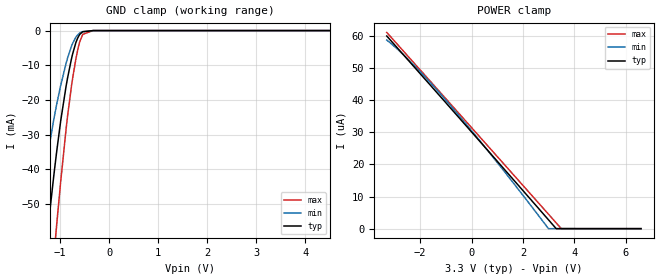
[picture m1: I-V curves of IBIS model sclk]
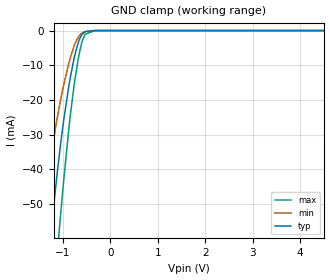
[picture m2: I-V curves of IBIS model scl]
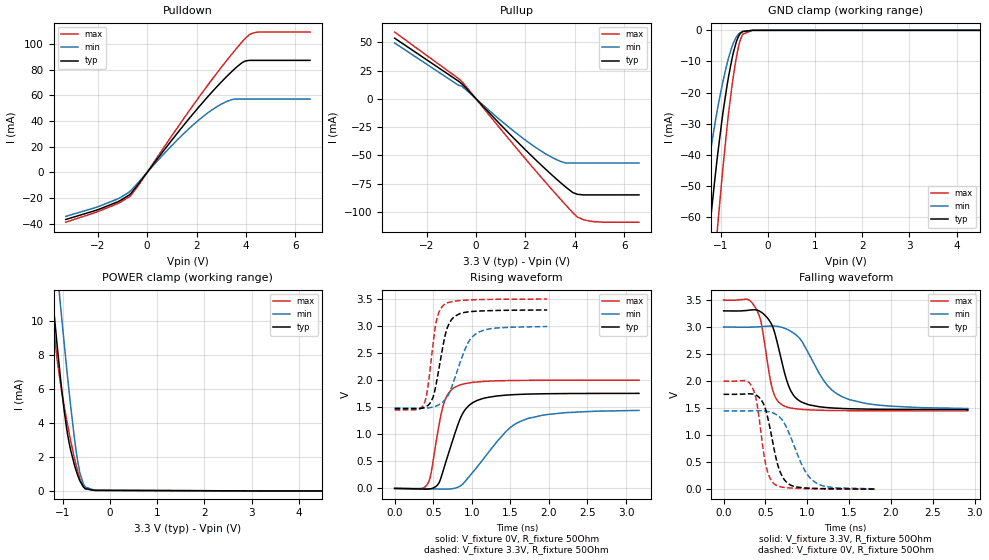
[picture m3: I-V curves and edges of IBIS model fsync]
|Texas Instruments Incorporated
|50-W, 2-MHz Digital Input 4-Channel Automotive Class-D Audio Amplifier
|With Load Dump Protection and I2C Diagnostics
|Marketing part#   Digital Voltage Range   Package-type   #pins
|TAS6424-Q1   3V - 26.4V   HSSOP   56
[IBIS Ver]   4.1
[File name]   tas6424_q1.ibs
[File Rev]   1.0
[Date]   9/17/2016
[Source]
| Texas Instruments Incorporated.
| Analog-eLab Design Center, HPA
| 12500 TI Blvd
| Dallas, TX -75243
[Notes]   Revision History:
| Rev 1.0: 9/17/2016
| - Initial version of the model
| - Model generated from simulations in SPECTRE
| - Model matched to SPICE simulation
| - C_comp although listed in numerical order of value are
|   obtained from varying PVT conditions. For PVT conditions for
|   each specific value refer the buffer description under
|   respective [Model]. IBIS model user is responsible for using
|   appropriate C_comp to simulate for Signal Integrity.
[Disclaimer]
| This model is designed as an aid for customers of Texas Instruments.
| TI and its licensors and suppliers make no warranties, either expressed
| or implied, with respect to this  model, including the warranties of
| merchantability or fitness for a particular purpose. The model is
| provided solely on an "as is" basis. The entire risk as to its quality
| and performance is with the customer.
[Copyright]
(C) Copyright 2016 Texas Instruments Incorporated.All rights reserved.
|   TAS6424_Q1DKQ
[Component]   TAS6424_Q1DKQ
[Manufacturer]   TI
[Package]   |56 DKQ - HSSOP Package
|   typ   min   max
R_pkg   0.2   0.16   0.24
L_pkg   1.5nH   1.2nH   1.8nH
C_pkg   0.4pF   0.32pF   0.48pF
[Pin]  signal_name   model_name   R_pin   L_pin   C_pin
1   GND   gnd   NA   NA   NA
2   PVDD   power   NA   NA   NA
3   VBAT   power   NA   NA   NA
4   AREF   power   NA   NA   NA
5   VREG   power   NA   NA   NA
6   VCOM   power   NA   NA   NA
7   AVSS   power   NA   NA   NA
8   AVDD   power   NA   NA   NA
9   GVDD   power   NA   NA   NA
10   GVDD   power   NA   NA   NA
11   GND   gnd   NA   NA   NA
12   MCLK   sclk   NA   NA   NA
13   SCLK   sclk   NA   NA   NA
14   FSYNC   fsync   NA   NA   NA
15   SDIN1   sclk   NA   NA   NA
16   SDIN2   sclk   NA   NA   NA
17   GND   gnd   NA   NA   NA
18   GND   gnd   NA   NA   NA
19   VDD   power   NA   NA   NA
20   SCL   scl   NA   NA   NA
21   SDA   sda   NA   NA   NA
22   I2C_ADDR0   fsync   NA   NA   NA
23   I2C_ADDR1   fsync   NA   NA   NA
24   _STANDBY   nc   NA   NA   NA
25   _MUTE   nc   NA   NA   NA
26   _FAULT   nc   NA   NA   NA
27   _WARN   nc   NA   NA   NA
28   GND   nc   NA   NA   NA
29   PVDD   power   NA   NA   NA
30   PVDD   power   NA   NA   NA
31   BST_1M   power   NA   NA   NA
32   OUT_1M   nc   NA   NA   NA
33   GND   gnd   NA   NA   NA
34   OUT_1P   nc   NA   NA   NA
35   BST_1P   power   NA   NA   NA
36   GND   gnd   NA   NA   NA
37   BST_2M   power   NA   NA   NA
38   OUT_2M   nc   NA   NA   NA
39   GND   gnd   NA   NA   NA
40   OUT_2P   nc   NA   NA   NA
41   BST_2P   power   NA   NA   NA
42   PVDD   power   NA   NA   NA
43   PVDD   power   NA   NA   NA
44   BST_3M   power   NA   NA   NA
45   OUT_3M   nc   NA   NA   NA
46   GND   gnd   NA   NA   NA
47   OUT_3P   nc   NA   NA   NA
48   BST_3P   power   NA   NA   NA
49   GND   gnd   NA   NA   NA
50   BST_4M   power   NA   NA   NA
51   OUT_4M   nc   NA   NA   NA
52   GND   gnd   NA   NA   NA
53   OUT_4P   nc   NA   NA   NA
54   BST_4P   power   NA   NA   NA
55   PVDD   power   NA   NA   NA
56   PVDD   power   NA   NA   NA
57   ThermalPad   gnd   NA   NA   NA
| Models and submodels in the file (4): sclk (Input), scl (Input), fsync (I/O), sda (I/O_open_drain)
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|   sclk Model
[Model]   sclk
Model_type   Input
Vinl = 0.99
Vinh = 2.31
|   typ   min   max
|   (nom PVT)   (fast PVT)   (slow PVT)
C_comp   6.288e-13   4.758e-13   7.537e-13
| Where nom  PVT is Nominal Process, 3.3V, 27C
|   Fast PVT is Strong Process,  3.5V, -40C
|   Slow PVT is Weak Process,   3V, 150C
[Model spec]
|subparameter
Vinl   0.99   0.90   1.05
Vinh   2.31   2.10   2.45
[Voltage Range]   3.3   3   3.5
|Junction Temperature
[Temperature Range]   27   150   -40
[Power Clamp Reference]   3.3   3   3.5
[GND Clamp Reference]   0   0   0
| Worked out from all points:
|   GND clamp passes 1 mA (typ) near -0.59 V on its own axis
[GND Clamp]
|   Voltage   I(typ)   I(min)   I(max)
-3.3V     -394.6mA   -304mA     -465.7mA
-1.544V   -99.89mA   -64.75mA   -138.1mA
-1.449V   -85.57mA   -54.72mA   -120.8mA
-1.287V   -62.45mA   -39.03mA   -92.13mA
-1.238V   -55.77mA   -34.62mA   -83.61mA
-1.105V   -39.1mA    -23.91mA   -61.71mA
-1.067V   -34.61mA   -21.1mA    -55.6mA
-877.8mV  -16.02mA   -9.455mA   -28.4mA
-769.5mV  -8.244mA   -4.559mA   -16.14mA
-642mV    -2.163mA   -1.241mA   -5.637mA
-538.5mV  -332.8uA   -295.2uA   -1.103mA
6.6V      0A         0A         0A
[POWER Clamp]
|   Voltage   I(typ)   I(min)   I(max)
-3.3V     59.92uA    58.65uA    61.04uA
-2.808V   55.49uA    55.28uA    56.63uA
-2.225V   50.24uA    50.72uA    51.41uA
-1.455V   43.28uA    44.1uA     44.5uA
-801mV    37.36uA    38.12uA    38.63uA
1.005V    20.95uA    20.55uA    22.41uA
2.997V    2.746uA    0A         4.496uA
3.297V    0A         0A         1.799uA
3.495V    0A         0A         17.75nA
6.6V      0A         0A         0A
|   scl Model
[Model]   scl
Model_type   Input
Vinl = 0.99
Vinh = 2.31
|   typ   min   max
|   (nom PVT)   (fast PVT)   (slow PVT)
C_comp   6.288e-13   4.758e-13   7.537e-13
| Where nom  PVT is Nominal Process, 3.3V, 27C
|   Fast PVT is Strong Process,  3.5V, -40C
|   Slow PVT is Weak Process,   3V, 150C
[Model spec]
|subparameter
Vinl   0.99   0.90   1.05
Vinh   2.31   2.10   2.45
[Voltage Range]   3.3   3   3.5
|Junction Temperature
[Temperature Range]   27   150   -40
[Power Clamp Reference]   3.3   3   3.5
[GND Clamp Reference]   0   0   0
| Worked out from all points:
|   GND clamp passes 1 mA (typ) near -0.59 V on its own axis
[GND Clamp]
|   Voltage   I(typ)   I(min)   I(max)
-3.3V     -394.6mA   -304mA     -465.7mA
-1.544V   -99.89mA   -64.75mA   -138.1mA
-1.449V   -85.57mA   -54.72mA   -120.8mA
-1.287V   -62.45mA   -39.03mA   -92.13mA
-1.238V   -55.77mA   -34.62mA   -83.61mA
-1.105V   -39.09mA   -23.91mA   -61.71mA
-1.067V   -34.61mA   -21.1mA    -55.6mA
-877.8mV  -16.02mA   -9.452mA   -28.4mA
-769.5mV  -8.242mA   -4.556mA   -16.14mA
-642mV    -2.16mA    -1.238mA   -5.635mA
-538.5mV  -329.1uA   -291.4uA   -1.101mA
6.6V      0A         0A         0A
[POWER Clamp]
|   Voltage   I(typ)   I(min)   I(max)
-3.3V     0A         0A         0A
0V        0A         0A         0A
6.6V      0A         0A         0A
|   fsync Model
[Model]   fsync
Model_type   I/O
Polarity   Non-Inverting
Enable   Active-High
Vinl = 0.99
Vinh = 2.31
Vmeas = 1.65
Vref = 0
Cref = 2pF
Rref = 70
|   typ   min   max
|   (nom PVT)   (fast PVT)   (slow PVT)
C_comp   9.736e-13   8.094e-13   1.100e-12
| Where nom  PVT is Nominal Process, 3.3V, 27C
|   Fast PVT is Strong Process,  3.5V, -40C
|   Slow PVT is Weak Process,   3V, 150C
[Model spec]
|subparameter
Vinl   0.99   0.90   1.05
Vinh   2.31   2.10   2.45
[Voltage Range]   3.3   3   3.5
|Junction Temperature
[Temperature Range]   27   150   -40
[Pullup Reference]   3.3   3   3.5
[Pulldown Reference]   0   0   0
[Power Clamp Reference]   3.3   3   3.5
[GND Clamp Reference]   0   0   0
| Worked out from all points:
|   slope of the pulldown table from 0 to 0.495 V, typ, clamps not added: 39.4 ohm
|   slope of the pullup table from 0 to 0.495 V, typ, clamps not added: 43.1 ohm
|   GND clamp passes 1 mA (typ) near -0.58 V on its own axis
|   POWER clamp passes 1 mA (typ) near -0.70 V on its own axis
|   falling waveform, V_fixture 3.3V, R_fixture 50Ohm: 20-80 % time 195ps typ, 378ps min, 135ps max; typ from 3.3 V to 1.47 V
|   rising waveform, V_fixture 0V, R_fixture 50Ohm: 20-80 % time 257ps typ, 519ps min, 157ps max; typ from 0 V to 1.76 V
|   rising waveform, V_fixture 3.3V, R_fixture 50Ohm: 20-80 % time 149ps typ, 236ps min, 112ps max; typ from 1.47 V to 3.3 V
|   falling waveform, V_fixture 0V, R_fixture 50Ohm: 20-80 % time 154ps typ, 245ps min, 115ps max; typ from 1.76 V to 0.004 V
[Pulldown]
|   Voltage   I(typ)   I(min)   I(max)
-3.3V     -36.59mA   -34.16mA   -38.69mA
-2.079V   -29.49mA   -27.22mA   -31.04mA
-1.203V   -22.91mA   -20.65mA   -24.25mA
-647mV    -16.03mA   -13.82mA   -17.58mA
994.5mV   25.05mA    20.91mA    28.46mA
2.373V    57.15mA    45.17mA    65.81mA
2.988V    70.06mA    53mA       81.42mA
3.408V    78.14mA    56.54mA    91.58mA
3.849V    85.46mA    57.07mA    101.7mA
4.143V    87.2mA     57.07mA    107.1mA
4.481V    87.2mA     57.07mA    109.2mA
6.6V      87.2mA     57.07mA    109.2mA
[GND Clamp]
|   Voltage   I(typ)   I(min)   I(max)
-3.3V     -440mA     -341.7mA   -519.1mA
-1.534V   -111.5mA   -73.85mA   -152.9mA
-1.431V   -94.25mA   -61.6mA    -132.1mA
-1.227V   -62.33mA   -39.69mA   -92.37mA
-1.062V   -39.41mA   -24.68mA   -62.25mA
-975mV    -28.86mA   -17.95mA   -47.56mA
-867.9mV  -17.84mA   -10.78mA   -31.2mA
-762.5mV  -9.177mA   -5.256mA   -17.88mA
-633mV    -2.229mA   -1.378mA   -5.882mA
-538.5mV  -388.1uA   -364.3uA   -1.272mA
-330mV    -4.25uA    -9.019uA   -5.089uA
6.6V      0A         0A         0A
[Pullup]
|   Voltage   I(typ)   I(min)   I(max)
-3.3V     53.6mA     49.34mA    59.01mA
-724mV    15.74mA    12.1mA     18.05mA
-588mV    13.44mA    11.21mA    15.53mA
1.284V    -29.46mA   -24.34mA   -34.44mA
2.553V    -56.88mA   -45.07mA   -67.28mA
2.973V    -65.43mA   -50.65mA   -77.83mA
3.51V     -75.83mA   -56.07mA   -91.03mA
3.901V    -82.68mA   -56.8mA    -100.4mA
4.095V    -84.42mA   -56.8mA    -104.4mA
4.353V    -85.03mA   -56.8mA    -107mA
4.795V    -85.03mA   -56.8mA    -108.7mA
6.6V      -85.03mA   -56.8mA    -109.2mA
[POWER Clamp]
|   Voltage   I(typ)   I(min)   I(max)
-3.3V     78.62mA    81.34mA    82.98mA
-1.294V   13.67mA    18.15mA    12.46mA
-1.224V   11.54mA    16.02mA    10.33mA
-1.123V   8.586mA    13.02mA    7.731mA
-1.056V   6.746mA    11.05mA    6.397mA
-976.8mV  4.8mA      8.789mA    5.06mA
-871mV    2.867mA    5.898mA    3.45mA
-696mV    993.8uA    1.895mA    1.238mA
-636.5mV  569.5uA    1.011mA    691.4uA
-525mV    128.3uA    227.9uA    131.5uA
-264mV    32.56uA    34.05uA    33.82uA
6.6V      0A         0A         0A
[Ramp]
R_load = 50
|   typ   min   max
dV/dt_r   1.05398/2.56961e-10   0.869396/5.22864e-10   1.20008/1.57028e-10
dV/dt_f   1.09538/1.94389e-10   0.908068/3.80996e-10   1.2297/1.34491e-10
[Falling Waveform]
V_fixture = 3.3V
V_fixture_min = 3V
V_fixture_max = 3.5V
R_fixture = 50Ohm
|   Time   V(typ)   V(min)   V(max)
0s        3.3V       3V         3.5V
281.6ps   3.308V     2.998V     3.519V
382.7ps   3.32V      3.002V     3.358V
452.5ps   3.275V     3.009V     3.06V
590ps     2.996V     3.02V      1.822V
729.9ps   2.15V      2.979V     1.537V
909.1ps   1.634V     2.791V     1.481V
1.197ns   1.517V     2.013V     1.46V
1.428ns   1.494V     1.704V     1.455V
2.92ns    1.474V     1.494V     1.45V
[Rising Waveform]
V_fixture = 0V
V_fixture_min = 0V
V_fixture_max = 0V
R_fixture = 50Ohm
|   Time   V(typ)   V(min)   V(max)
0s        345.2pV    23.28nV    146.2pV
432.7ps   -12.69mV   -4.635mV   96.19mV
471.2ps   -5.458mV   -6.65mV    271.6mV
564.5ps   79.77mV    -11.33mV   1.087V
644.3ps   400.1mV    -13.85mV   1.602V
816.8ps   1.164V     20.23mV    1.894V
919.8ps   1.465V     140.5mV    1.938V
1.062ns   1.621V     383.8mV    1.966V
1.635ns   1.738V     1.242V     1.995V
3.168ns   1.756V     1.441V     2V
[Rising Waveform]
V_fixture = 3.3V
V_fixture_min = 3V
V_fixture_max = 3.5V
R_fixture = 50Ohm
|   Time   V(typ)   V(min)   V(max)
0s        1.474V     1.486V     1.45V
382.7ps   1.495V     1.481V     1.569V
429ps     1.531V     1.487V     1.856V
496.4ps   1.679V     1.504V     2.646V
540ps     1.94V      1.524V     3.083V
647.9ps   2.784V     1.629V     3.401V
771.7ps   3.171V     2.003V     3.458V
911.6ps   3.253V     2.567V     3.477V
1.039ns   3.272V     2.841V     3.485V
1.977ns   3.297V     2.991V     3.498V
[Falling Waveform]
V_fixture = 0V
V_fixture_min = 0V
V_fixture_max = 0V
R_fixture = 50Ohm
|   Time   V(typ)   V(min)   V(max)
0s        1.757V     1.449V     2V
346ps     1.763V     1.452V     1.876V
399.8ps   1.733V     1.454V     1.584V
510ps     1.438V     1.445V     416.5mV
616.5ps   649mV      1.394V     86.83mV
681.2ps   303.6mV    1.319V     46.63mV
765.1ps   113mV      1.1V       27.92mV
972.2ps   25.29mV    342mV      13.23mV
1.087ns   16.68mV    137mV      9.613mV
1.817ns   3.697mV    8.046mV    2.24mV
